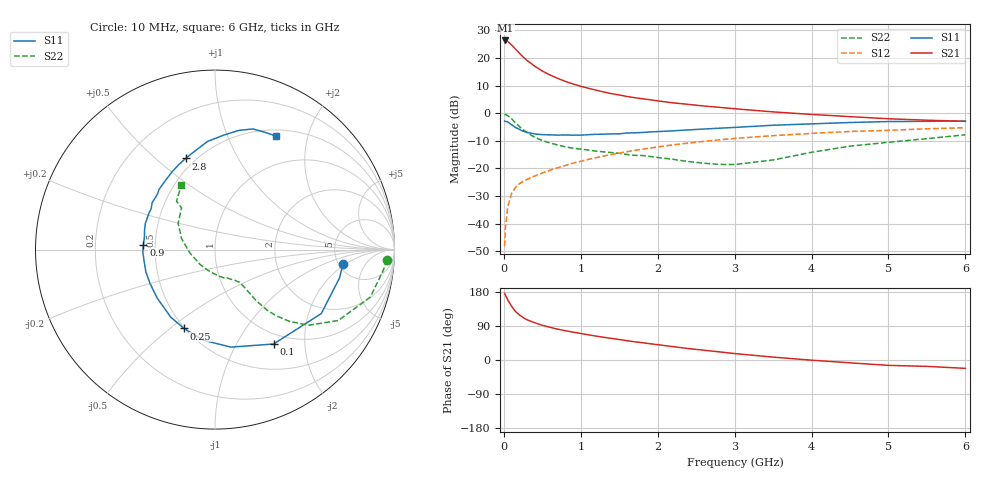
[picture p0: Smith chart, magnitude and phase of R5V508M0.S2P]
! SIEMENS Small Signal Semiconductors
! BFR183
! Si NPN RF Bipolar Junction Transistor in SOT23
! VCE = 0.5 V  IC = 8 mA
! Common Emitter S-Parameters:  May  1996
# GHz  S  MA  R  50
!  f  S11  S21  S12  S22
! GHz  MAG  ANG  MAG  ANG  MAG  ANG  MAG  ANG
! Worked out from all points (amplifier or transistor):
!   36 points, 10 MHz to 6 GHz, reference 50 ohm
!   highest |S21| = 26.3 dB at 20 MHz (marker M1)
!   |S21| within 3 dB of that: start of sweep to 146.4 MHz
!   unconditionally stable (mu >= 1): 686.7 MHz to 3.496 GHz
!   at 250 MHz: K = 0.59, MSG = 22.5 dB, |S12| = -24.7 dB
!   at 1.4 GHz: K = 1.11, MAG = 9.0 dB, |S12| = -15.0 dB
!   at 6 GHz: K = 0.98, MSG = 1.2 dB, |S12| = -5.3 dB
!   S11 on the Smith chart (normalised r, x): 10 MHz: 5.42, -1.84; 100 MHz: 0.84, -1.44; 250 MHz: 0.50, -0.56; 900 MHz: 0.43, +0.03; 2.8 GHz: 0.44, +0.63; 6 GHz: 0.58, +1.52
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0.01  0.717 -6.6  20.62 175.9  0.0039 86.5  0.9589 -3.4
0.02  0.7117 -12.8  20.71 171.1  0.0082 85.4  0.9449 -7.0
0.05  0.691 -31.1  19.85 159.1  0.0199 75.8  0.905 -17.0
0.1  0.6189 -58.2  17.21 142.2  0.0349 65.2  0.7923 -29.9
0.15  0.5506 -80.7  14.48 128.4  0.0449 58.3  0.6699 -39.0
0.2  0.5093 -97.2  12.26 119.4  0.0524 54.7  0.5754 -44.0
0.25  0.4722 -111.5  10.42 112.0  0.0582 53.2  0.5024 -47.2
0.3  0.4498 -123.3  9.036 106.4  0.0631 53.1  0.4453 -49.3
0.4  0.4203 -140.1  7.11 98.3  0.0727 53.5  0.3666 -51.1
0.5  0.4082 -152.6  5.787 91.7  0.0823 54.3  0.3187 -51.5
0.6  0.4047 -162.3  4.911 86.2  0.0926 55.1  0.2885 -51.8
0.7  0.3999 -171.3  4.27 81.4  0.1023 55.9  0.2646 -52.1
0.9  0.3998 176.0  3.372 73.5  0.1244 56.8  0.2315 -52.9
1.1  0.4071 164.5  2.82 66.5  0.1454 56.4  0.2148 -55.5
1.3  0.4165 155.1  2.417 59.9  0.1676 55.4  0.1988 -58.0
1.6  0.4368 143.3  2.002 50.9  0.2005 53.3  0.1785 -64.5
2.2  0.4782 124.0  1.536 35.3  0.2665 47.3  0.1457 -84.2
2.8  0.5337 107.8  1.275 21.5  0.3284 39.9  0.118 -119.3
3.5  0.6039 94.0  1.054 7.6  0.391 30.0  0.1421 -173.1
4.5  0.6768 78.8  0.865 -7.4  0.4658 16.7  0.2524 144.5
5.5  0.7109 66.5  0.745 -16.8  0.5206 5.5  0.345 128.4
6  0.7182 61.6  0.712 -22.1  0.544 -1.8  0.4061 117.5
